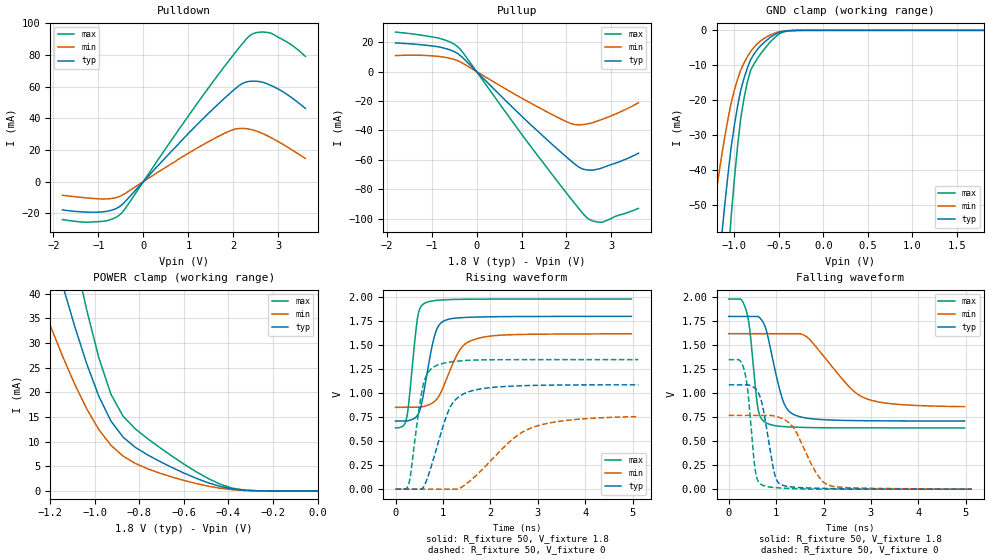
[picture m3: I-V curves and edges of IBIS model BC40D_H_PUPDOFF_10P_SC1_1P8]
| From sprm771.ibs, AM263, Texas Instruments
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|   Model Cell BC40D_H_PUPDOFF_10P_SC1_1P8
|BC40D_H_PUPDOFF_10P_SC1_1P8
[Model]   BC40D_H_PUPDOFF_10P_SC1_1P8
Model_type   I/O
Polarity   Non-Inverting
Enable   Active-Low
Vinl =  0.63
Vinh =  1.17
Cref =  15pF
Rref =  100.0000M
Vref =  0V
Vmeas =  0.9
C_comp   2.389419p   2.292106p   2.408415p
|[Input load] weak_pupdoff
|[Output drive] slow
|[supplytol] 10
|[temp] ind
[Model Spec]
Vinl   0.63   0.567   0.693
Vinh   1.17   1.053   1.287
[Temperature Range]   25   125   -40
[Voltage Range]   1.8   1.62   1.98
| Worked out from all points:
|   slope of the pulldown table from 0 to 0.27 V, typ, clamps not added: 32.2 ohm
|   slope of the pullup table from 0 to 0.27 V, typ, clamps not added: 32.6 ohm
|   GND clamp passes 1 mA (typ) near -0.53 V on its own axis
|   POWER clamp passes 1 mA (typ) near -0.44 V on its own axis
|   rising waveform, R_fixture 50, V_fixture 1.8: 20-80 % time 249ps typ, 424ps min, 162ps max; typ from 0.709 V to 1.8 V
|   rising waveform, R_fixture 50, V_fixture 0: 20-80 % time 430ps typ, 994ps min, 232ps max; typ from 0 V to 1.09 V
|   falling waveform, R_fixture 50, V_fixture 1.8: 20-80 % time 310ps typ, 792ps min, 166ps max; typ from 1.8 V to 0.709 V
|   falling waveform, R_fixture 50, V_fixture 0: 20-80 % time 228ps typ, 466ps min, 151ps max; typ from 1.09 V to 0 V
| Nom Voltages:
|   VDD=1.1001, VDDS=1.8, VDDS18=1.8, ESD_BIASFET=0, VSS=0, VSSS=0
| Min Voltages:
|   VDD=0.99, VDDS=1.62, VDDS18=1.62, ESD_BIASFET=0, VSS=0, VSSS=0
| Max Voltages:
|   VDD=1.21, VDDS=1.98, VDDS18=1.98, ESD_BIASFET=0, VSS=0, VSSS=0
[POWER_clamp]
|   voltage   I(typ)   I(min)   I(max)
-1.8V     158.8mA    112.5mA    219.7mA
-1.255V   59.93mA    40mA       84.85mA
-1.127V   39.08mA    25.51mA    55.74mA
-1.055V   28.36mA    18.34mA    40.4mA
-981.8mV  19.18mA    12.43mA    26.97mA
-927.3mV  14.16mA    9.242mA    19.58mA
-872.7mV  10.89mA    7.052mA    15.14mA
-818.2mV  8.843mA    5.581mA    12.58mA
-600mV    3.63mA     2.129mA    5.448mA
-436.4mV  903.9uA    539.1uA    1.358mA
-327.3mV  138.2uA    94.86uA    160.4uA
0V        19.3nA     120.3nA    352.8nA
[Pulldown]
|   voltage   I(typ)   I(min)   I(max)
-1.8V     -17.92mA   -8.674mA   -24.03mA
-927.3mV  -19.22mA   -10.99mA   -25.2mA
-654.5mV  -17.65mA   -10.46mA   -23.22mA
-490.9mV  -14.97mA   -8.904mA   -20.12mA
872.7mV   26.63mA    15.72mA    36.29mA
1.691V    49.7mA     28.87mA    68.59mA
2.127V    60.63mA    33.53mA    84.59mA
2.4V      63.43mA    32.84mA    92.9mA
2.618V    62.99mA    30.74mA    94.47mA
2.836V    60.69mA    27.76mA    93.76mA
3.273V    53.49mA    20.53mA    86.73mA
3.6V      46.26mA    14.64mA    79.12mA
[Pullup]
|   voltage   I(typ)   I(min)   I(max)
-1.8V     19.42mA    10.82mA    26.76mA
-818.2mV  16.58mA    10.15mA    22.47mA
-545.5mV  14.19mA    8.648mA    19.37mA
-381.8mV  11.34mA    6.842mA    15.75mA
1.036V    -31.26mA   -18.6mA    -43.9mA
1.909V    -55.59mA   -32.73mA   -78.89mA
2.182V    -62.72mA   -35.92mA   -89.47mA
2.345V    -65.94mA   -36.05mA   -95.62mA
2.455V    -66.75mA   -35.58mA   -99.18mA
2.618V    -66.67mA   -34.29mA   -101.7mA
2.782V    -65.46mA   -32.56mA   -102.2mA
3.6V      -55.4mA    -21.22mA   -92.82mA
[GND_clamp]
|   voltage   I(typ)   I(min)   I(max)
-1.8V     -270.2mA   -170.2mA   -430.1mA
-1.255V   -91.66mA   -55.91mA   -148.4mA
-1.145V   -59.91mA   -36.44mA   -97.09mA
-1.109V   -50.48mA   -30.83mA   -81.55mA
-1.073V   -41.73mA   -25.65mA   -67.05mA
-1.036V   -33.66mA   -20.92mA   -53.59mA
-927.3mV  -17.07mA   -11.35mA   -25.04mA
-854.5mV  -10.86mA   -7.616mA   -14.91mA
-781.8mV  -6.919mA   -4.945mA   -9.771mA
-636.4mV  -2.823mA   -1.868mA   -4.529mA
-381.8mV  -84.73uA   -78.7uA    -126.1uA
1.8V      19.3nA     3.129uA    310.3nA
[Ramp]
| variable   typ   min   max
dV/dt_f 0.66158688/0.31325875n 0.46775991/0.81492844n 0.81092193/0.16803896n
dV/dt_r 0.65950975/0.4332659n 0.47445273/1.0528319n 0.81583137/0.23271255n
R_load = 50
[Rising Waveform]
R_fixture = 50
V_fixture = 1.8
V_fixture_min = 1.62
V_fixture_max = 1.98
|   time   V(typ)   V(min)   V(max)
0s        709.1mV    852.1mV    638.7mV
228.1ps   709.1mV    852.1mV    727.1mV
278.6ps   715mV      852.1mV    897mV
460.2ps   767.3mV    852.4mV    1.774V
614.5ps   1.062V     864mV      1.936V
841.9ps   1.628V     923mV      1.965V
1.074ns   1.764V     1.146V     1.974V
1.389ns   1.786V     1.472V     1.978V
1.776ns   1.794V     1.576V     1.979V
4.974ns   1.8V       1.618V     1.98V
[Rising Waveform]
R_fixture = 50
V_fixture = 0
V_fixture_min = 0
V_fixture_max = 0
|   time   V(typ)   V(min)   V(max)
0s        0V         0V         0V
273.6ps   0V         0V         47.5mV
574.1ps   10.47mV    0V         1.068V
678.9ps   125.1mV    0V         1.21V
834.8ps   374mV      0V         1.281V
1.162ns   862.8mV    0V         1.325V
1.553ns   1.016V     78.35mV    1.343V
2.437ns   1.073V     507.6mV    1.349V
2.86ns    1.08V      637.5mV    1.349V
5.123ns   1.087V     755.3mV    1.349V
[Falling Waveform]
R_fixture = 50
V_fixture = 1.8
V_fixture_min = 1.62
V_fixture_max = 1.98
|   time   V(typ)   V(min)   V(max)
0s        1.799V     1.619V     1.98V
369ps     1.799V     1.619V     1.862V
442ps     1.799V     1.619V     1.673V
616.5ps   1.799V     1.619V     845.8mV
787.4ps   1.665V     1.619V     691.7mV
1.132ns   939.8mV    1.619V     652.6mV
1.381ns   775.6mV    1.619V     645.7mV
1.677ns   737.5mV    1.574V     641.7mV
2.853ns   712.9mV    951.9mV    638.2mV
4.974ns   709mV      859.5mV    637.9mV
[Falling Waveform]
R_fixture = 50
V_fixture = 0
V_fixture_min = 0
V_fixture_max = 0
|   time   V(typ)   V(min)   V(max)
0s        1.086V     768.8mV    1.348V
333.6ps   1.086V     768.8mV    1.229V
404.9ps   1.086V     768.8mV    1.016V
557ps     1.051V     768.8mV    209.4mV
685.7ps   926.1mV    768.8mV    47.75mV
959.6ps   176mV      762.7mV    16.78mV
1.118ns   44.32mV    737.9mV    11.66mV
1.37ns    20.88mV    639mV      5.036mV
2.109ns   6.098mV    41.68mV    0V
5.123ns   0V         2.126mV    0V
